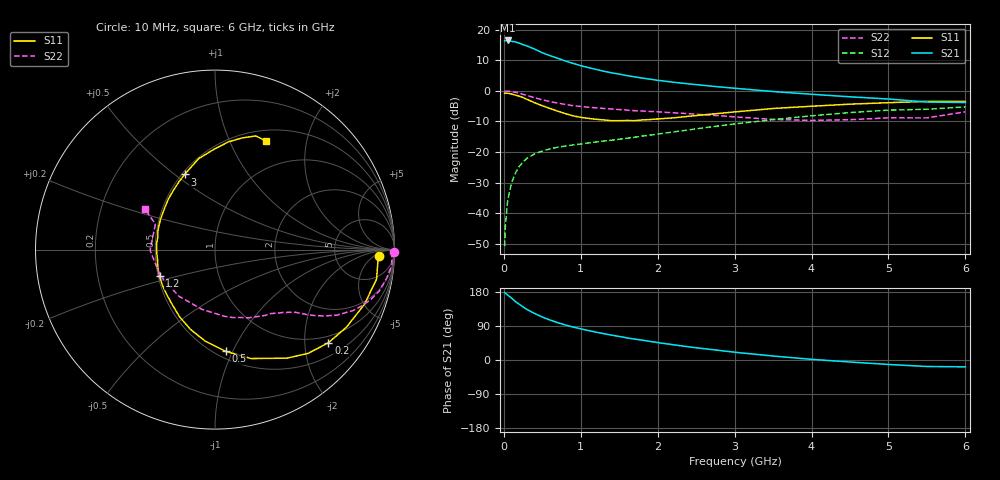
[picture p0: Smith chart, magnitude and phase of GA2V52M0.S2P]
! Infineon Technologies  Discrete & RF Semiconductors
! BF775
! Si NPN RF Bipolar Junction Transistor in SOT23
! VCE = 2.5 V  IC = 2 mA
! Common Emitter S-Parameters:  May  1996
# GHz  S  MA  R  50
!  f  S11  S21  S12  S22
! GHz  MAG  ANG  MAG  ANG  MAG  ANG  MAG  ANG
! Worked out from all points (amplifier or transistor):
!   36 points, 10 MHz to 6 GHz, reference 50 ohm
!   highest |S21| = 16.5 dB at 50 MHz (marker M1)
!   |S21| within 3 dB of that: start of sweep to 414.8 MHz
!   unconditionally stable (mu >= 1): 1.155 GHz to 4.101 GHz; 5.188 GHz to end of sweep
!   at 250 MHz: K = 0.28, MSG = 19.1 dB, |S12| = -23.2 dB
!   at 1.4 GHz: K = 1.11, MAG = 9.0 dB, |S12| = -16.1 dB
!   at 6 GHz: K = 1.01, MAG = 0.3 dB, |S12| = -5.2 dB
!   S11 on the Smith chart (normalised r, x): 10 MHz: 19, -8; 200 MHz: 0.82, -2.56; 500 MHz: 0.56, -0.94; 1.2 GHz: 0.51, -0.17; 3 GHz: 0.52, +0.54; 6 GHz: 0.63, +1.38
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0.01  0.9145 -2.1  6.522 178.6  0.0029 88.4  0.9976 -0.9
0.02  0.91 -4.1  6.598 176.4  0.0063 89.6  0.9855 -1.9
0.05  0.9152 -10.3  6.646 171.4  0.0162 83.0  0.9894 -4.9
0.1  0.8864 -20.2  6.43 163.4  0.0313 78.1  0.97 -9.4
0.15  0.8505 -30.5  6.301 154.3  0.0455 72.4  0.9448 -14.0
0.2  0.8176 -39.4  6.002 147.2  0.0582 67.7  0.9121 -17.7
0.3  0.7255 -56.5  5.407 133.4  0.079 59.5  0.841 -23.8
0.4  0.6393 -71.7  4.802 122.9  0.0932 53.8  0.7702 -28.3
0.5  0.5702 -83.9  4.184 113.3  0.1038 49.4  0.7117 -31.3
0.6  0.5139 -95.9  3.754 105.5  0.1127 46.7  0.668 -33.4
0.7  0.4654 -107.0  3.401 98.5  0.1198 44.7  0.6307 -35.1
0.8  0.4239 -117.7  3.069 92.4  0.1253 43.5  0.5986 -36.5
0.9  0.3898 -127.2  2.804 87.0  0.1306 43.0  0.5723 -37.7
1.1  0.3547 -145.5  2.395 77.7  0.1409 42.5  0.5395 -40.3
1.2  0.3429 -154.3  2.234 73.4  0.1458 42.4  0.5267 -41.7
1.6  0.3276 174.5  1.77 58.4  0.168 44.1  0.4838 -47.2
2.2  0.3614 141.6  1.383 40.3  0.2127 45.4  0.4378 -58.8
3  0.4519 112.0  1.102 20.5  0.2877 42.2  0.3755 -81.8
3.5  0.5146 100.2  0.973 10.5  0.3384 37.7  0.341 -102.2
4.5  0.6054 82.8  0.798 -5.3  0.4413 25.5  0.3375 -154.7
5.5  0.6724 70.3  0.655 -17.1  0.4998 9.9  0.3612 156.9
6  0.6694 65.0  0.644 -18.1  0.5465 5.6  0.4534 149.7
